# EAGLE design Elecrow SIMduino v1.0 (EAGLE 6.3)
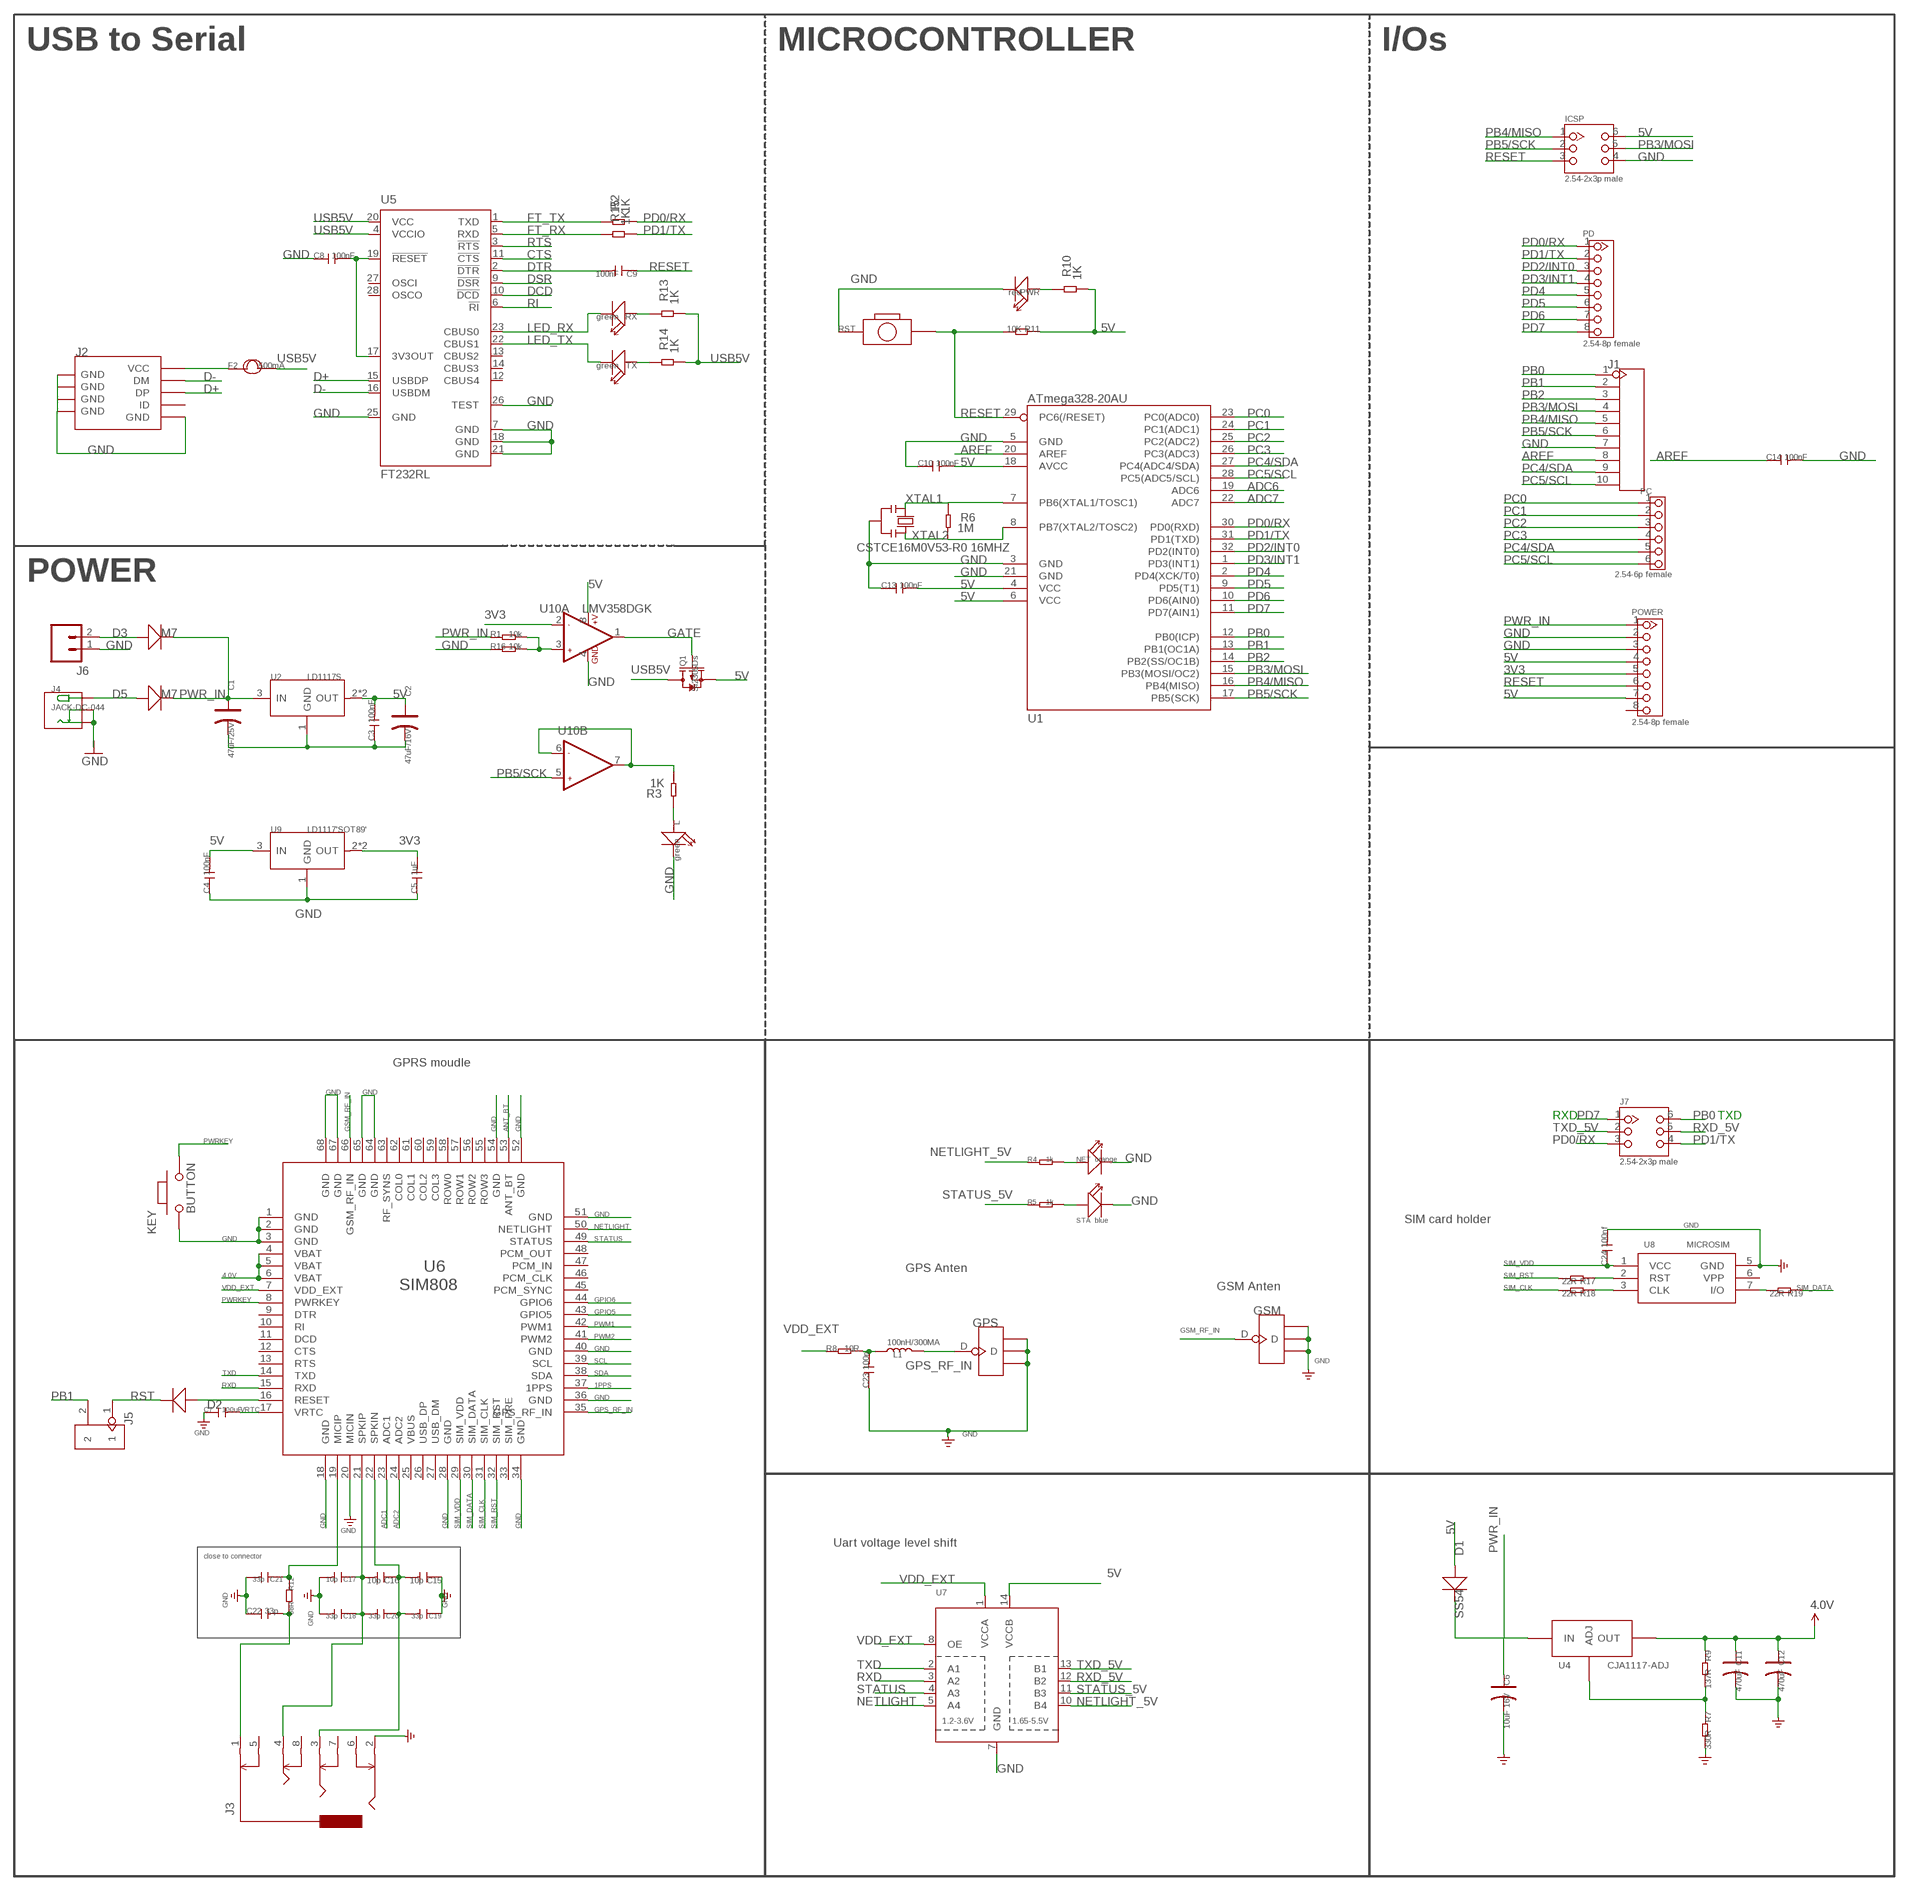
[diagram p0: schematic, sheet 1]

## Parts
C1  47uF/25V  CAP-AVX-C  [AVX-C]
C2  47uF/16V  CAP-AVX-A  [AVX-A]
C3  100nF  C-0603  [C0603]
C4  100nF  C-0603  [C0603]
C5  1uF  C-0603  [C0603]
C6  10uF 16V  CAP-AVX-A  [AVX-A]
C7  100uF  C-0805  [C0805]
C8  100nF  C-0603  [C0603]
C9  100nF  C-0603  [C0603]
C10  100nF  C-0603  [C0603]
C11  470uF  CAP-AVX-D  [AVX-D]
C12  470uF  CAP-AVX-D  [AVX-D]
C13  100nF  C-0603  [C0603]
C14  100nF  C-0603  [C0603]
C15  10p  C-0402  [C0402]
C16  10p  C-0402  [C0402]
C17  10p  C-0402  [C0402]
C18  33p  C-0402  [C0402]
C19  33p  C-0402  [C0402]
C20  33p  C-0402  [C0402]
C21  33p  C-0603  [C0603]
C22  33p  C-0603  [C0603]
C23  100n  C-0603  [C0603]
C24  100nf  C-0603  [C0603]
D1  SS54  D'MBRS240LT3'  [SMB]
D2  D'0805'  [SOD323]
D3  M7  D'SMA'  [D2010]
D5  M7  D'SMA'  [D2010]
F2  500mA  FUSE1206  [R1206]
GPS  ANTENNA-U-FL  [4P-U-FL]
GSM  ANTENNA-U-FL  [4P-U-FL]
ICSP  2.54-2x3p male  HEADER-2X3P-2.54  [2X3P-2.54]
J1  HEADER-10P-2.54  [10P-2.54]
J2  USB-MINIUSB-5P-STRONG  [MINI-SMD-5P]
J3  AUDIO-8P'PJ-3536-L6S'  [8P-3.5-SMD]
J4  JACK-DC-044  [DC-404]
J5  HEADER-2P-65/35MIL  [2P-2.54-65/35MIL]
J6  M02-JST-2MM-SMT  [JST-2-SMD]
J7  2.54-2x3p male  HEADER-2X3P-2.54  [2X3P-2.54]
KEY  BUTTON  PB157  [157SW]
L  green  LED'0603'  [LED-0603]
L1  100nH/300MA  L'0603'  [L0603]
NET  orange  LED'0603'  [LED-0603]
PC  2.54-6p female  HEADER-6P-65/35MIL  [6P-2.54-65/35MIL]
PD  2.54-8p female  HEADER-8P-2.54  [8P-2.54]
POWER  2.54-8p female  HEADER-8P-2.54  [8P-2.54]
PWR  red  LED'0603'  [LED-0603]
Q1  Si2305Ds  MOSFET-P'SI2323CDS/SI2305DS<BR>'  [SOT23]
R1  10k  R-0603  [R0603]
R2  1K  R-0603  [R0603]
R3  1K  R-0603  [R0603]
R4  1k  R-0603  [R0603]
R5  1k  R-0603  [R0603]
R6  1M  R-0603  [R0603]
R7  330R  R-0603  [R0603]
R8  10R  R-0603  [R0603]
R9  137R  R-0603  [R0603]
R10  1K  R-0603  [R0603]
R11  10K  R-0603  [R0603]
R12  68R  R-0603  [R0603]
R13  1K  R-0603  [R0603]
R14  1K  R-0603  [R0603]
R15  1K  R-0603  [R0603]
R16  10k  R-0603  [R0603]
R17  22R  R-0603  [R0603]
R18  22R  R-0603  [R0603]
R19  22R  R-0603  [R0603]
RST  BOTTON-2P-90D  [2P-7.62X3.56-90D]
RX  green  LED'0603'  [LED-0603]
STA  blue  LED'0603'  [LED-0603]
TX  green  LED'0603'  [LED-0603]
U1  ATmega328-20AU  ATMEGA168  [TQFP32]
U2  LD1117S  [SOT-223]
U4  CJA1117-ADJ  [SOT89]
U5  FT232RL  [SSOP28]
U6  SIM808  [SIM808]
U7  TXB0104PWR  [TSSOP14]
U8  MICROSIM  [MICROSIM]
U9  LD1117'SOT89'  [SOT89]
U10  LMV358DGK  [MSOP8]
Y2  CSTCE16M0V53-R0 16MHZ  RESONATORMU  [RESONATOR]

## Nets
1PPS: U6.37(1PPS)
3V3: C5.2 POWER.5 U9.2(OUT) U9.4(OUT) U10.2(A:-IN1)
4.0V: C11.+ C12.+ R9.1 U4.2(OUT) U4.4(OUT) U6.4(VBAT) U6.5(VBAT) U6.6(VBAT)
5V [usbvcc]: C2.+ C3.2 C4.2 C10.2 C13.2 D1.+ ICSP.6 POWER.4 POWER.7 Q1.2(S) R10.1 R11.1 U1.4(VCC) U1.6(VCC) U1.18(AVCC) U2.2(OUT) U2.TER(OUT) U7.14(VCCB) U9.3(IN) U10.8(A:+V)
ADC1: U6.23(ADC1)
ADC2: U6.24(ADC2)
ADC6: U1.19(ADC6)
ADC7: U1.22(ADC7)
ANT_BT: U6.53(ANT_BT)
AREF: C14.1 J1.8 U1.20(AREF)
CTS: U5.11(!CTS)
D+: J2.3(DP) U5.15(USBDP)
D-: J2.2(DM) U5.16(USBDM)
DCD: U5.10(!DCD)
DSR: U5.9(!DSR)
DTR: C9.2 U5.2(!DTR)
FT_RX: R15.2 U5.5(RXD)
FT_TX: R2.2 U5.1(TXD)
GATE: Q1.1(G) U10.1(A:OUT1)
GND: C1.- C2.- C3.1 C4.1 C5.1 C6.- C7.1 C8.1 C10.1 C11.- C12.- C13.1 C14.2 C15.1 C17.2 C18.2 C19.1 C21.2 C22.1 C23.1 C24.2 GPS.GND1 GPS.GND2 GPS.GND3 GSM.GND1 GSM.GND2 GSM.GND3 ICSP.4 J1.7 J2.5(GND) J2.GND@1(GND) J2.GND@2(GND) J2.GND@3(GND) J2.GND@4(GND) J3.2 J4.- J4.CDN J6.1 KEY.1 L.- NET.- POWER.2 POWER.3 PWR.- R7.2 R16.1 RST.P$1 STA.- U1.3(GND) U1.5(GND) U1.21(GND) U2.1(GND) U5.7(GND) U5.18(GND) U5.21(GND) U5.25(GND) U5.26(TEST) U6.1(GND) U6.2(GND) U6.3(GND) U6.18(GND) U6.20(MICIN) U6.28(GND) U6.34(GND) U6.36(GND) U6.40(GND) U6.51(GND) U6.52(GND) U6.54(GND) U6.64(GND) U6.65(GND) U6.67(GND) U6.68(GND) U7.7(GND) U8.5(GND) U9.1(GND) U10.4(A:GND) Y2.2
GPIO5: U6.43(GPIO5)
GPIO6: U6.44(GPIO6)
GPS_RF_IN: GPS.D L1.2 U6.35(GPS_RF_IN)
GSM_RF_IN: GSM.D U6.66(GSM_RF_IN)
LED_RX: RX.- U5.23(CBUS0)
LED_TX: TX.- U5.22(CBUS1)
N$1: D5.+ J4.+
N$2: R13.2 RX.+
N$3: L.+ R3.2
N$4: R5.2 STA.+
N$5: R3.1 U10.6(B:-IN2) U10.7(B:OUT2)
N$6: C8.2 U5.17(3V3OUT) U5.19(!RESET)
N$7: PWR.+ R10.2
N$8: R14.2 TX.+
N$9: F2.1 J2.1(VCC)
N$10: NET.+ R4.2
N$11: R18.1 U8.3(CLK)
N$12: R17.1 U8.2(RST)
N$13: C21.1 R12.1 U6.19(MICIP)
N$14: R1.2 R16.2 U10.3(A:+IN1)
N$15: C16.2 C17.1 C18.1 C20.2 J3.4 U6.21(SPKIP)
N$16: R19.2 U8.7(I/O)
N$17: R7.1 R9.2 U4.1(ADJ)
N$18: D2.+ U6.16(RESET)
N$19: C15.2 C16.1 C19.2 C20.1 J3.3 U6.22(SPKIN)
N$20: D3.+ J6.2
N$21: C23.2 L1.1 R8.2
N$30: C22.2 J3.1 R12.2
NETLIGHT: U6.50(NETLIGHT) U7.5(A4)
NETLIGHT_5V: R4.1 U7.10(B4)
PB0: J1.1 J7.6 U1.12(PB0(ICP))
PB1: J1.2 J5.2 U1.13(PB1(OC1A))
PB2: J1.3 U1.14(PB2(SS/OC1B))
PB3/MOSI: ICSP.5 J1.4 U1.15(PB3(MOSI/OC2))
PB4/MISO: ICSP.1 J1.5 U1.16(PB4(MISO))
PB5/SCK: ICSP.2 J1.6 U1.17(PB5(SCK)) U10.5(B:+IN2)
PC0: PC.1 U1.23(PC0(ADC0))
PC1: PC.2 U1.24(PC1(ADC1))
PC2: PC.3 U1.25(PC2(ADC2))
PC3: PC.4 U1.26(PC3(ADC3))
PC4/SDA: J1.9 PC.5 U1.27(PC4(ADC4/SDA))
PC5/SCL: J1.10 PC.6 U1.28(PC5(ADC5/SCL))
PD0/RX: J7.3 PD.1 R2.1 U1.30(PD0(RXD))
PD1/TX: J7.4 PD.2 R15.1 U1.31(PD1(TXD))
PD2/INT0: PD.3 U1.32(PD2(INT0))
PD3/INT1: PD.4 U1.1(PD3(INT1))
PD4: PD.5 U1.2(PD4(XCK/T0))
PD5: PD.6 U1.9(PD5(T1))
PD6: PD.7 U1.10(PD6(AIN0))
PD7: J7.1 PD.8 U1.11(PD7(AIN1))
PWM1: U6.42(PWM1)
PWM2: U6.41(PWM2)
PWR_IN: C1.+ C6.+ D1.- D3.- D5.- POWER.1 R1.1 U2.3(IN) U4.3(IN)
PWRKEY: KEY.2 U6.8(PWRKEY)
RESET: C9.1 ICSP.3 POWER.6 R11.2 RST.P$2 U1.29(PC6(/RESET))
RI: U5.6(!RI)
RST: D2.- J5.1
RTS: U5.3(!RTS)
RXD: U6.15(RXD) U7.3(A2)
RXD_5V: J7.5 U7.12(B2)
SCL: U6.39(SCL)
SDA: U6.38(SDA)
SIM_CLK: R18.2 U6.31(SIM_CLK)
SIM_DATA: R19.1 U6.30(SIM_DATA)
SIM_RST: R17.2 U6.32(SIM_RST)
SIM_VDD: C24.1 U6.29(SIM_VDD) U8.1(VCC)
STATUS: U6.49(STATUS) U7.4(A3)
STATUS_5V: R5.1 U7.11(B3)
TXD: U6.14(TXD) U7.2(A1)
TXD_5V: J7.2 U7.13(B1)
USB5V: F2.2 Q1.3(D) R13.1 R14.1 U5.4(VCCIO) U5.20(VCC)
VDD_EXT: R8.1 U6.7(VDD_EXT) U7.1(VCCA) U7.8(OE)
VRTC: C7.2 U6.17(VRTC)
XTAL1: R6.2 U1.7(PB6(XTAL1/TOSC1)) Y2.1
XTAL2: R6.1 U1.8(PB7(XTAL2/TOSC2)) Y2.3
Unconnected: J2.4(ID) J3.5 J3.6 J3.7 J3.8 POWER.8 U5.12(CBUS4) U5.13(CBUS2) U5.14(CBUS3) U5.27(OSCI) U5.28(OSCO) U6.9(DTR) U6.10(RI) U6.11(DCD) U6.12(CTS) U6.13(RTS) U6.25(VBUS) U6.26(USB_DP) U6.27(USB_DM) U6.33(SIM_PRE) U6.45(PCM_SYNC) U6.46(PCM_CLK) U6.47(PCM_IN) U6.48(PCM_OUT) U8.6(VPP)

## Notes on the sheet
- USB to Serial | MICROCONTROLLER | I/Os
- POWER
- GPRS moudle
- RXD | TXD
- SIM card holder
- GPS Anten
- GSM Anten
- Uart voltage level shift
- close to connector

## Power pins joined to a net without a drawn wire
COL0: U6.62(COL0)
COL1: U6.61(COL1)
COL2: U6.60(COL2)
COL3: U6.59(COL3)
RF_SYNS: U6.63(RF_SYNS)
ROW0: U6.58(ROW0)
ROW1: U6.57(ROW1)
ROW2: U6.56(ROW2)
ROW3: U6.55(ROW3)

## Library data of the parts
C1 C2 = Discrete:CAP*: Electrolytic Capacitors,Tantalum Capacitors and Super Capacitors
C3-C5 C7-C10 C13-C24 = Discrete:C*: Ceramic Capacitors
C6 C11 C12 = Common:CAP*
D1-D3 D5 = Discrete:D*
F2 = Discrete:FUSE
GPS GSM = Connector:ANTENNA-U-FL
ICSP J7 = Connector:HEADER-2X3P
J1 = Connector:HEADER-10P
J2 = Connector:USB-MINIUSB-5P
J3 = template:AUDIO-8P
J4 = Connector:JACK-DC-044
J5 = Connector:HEADER-2P
J6 = SparkFun:M02: Header 2
KEY = MySMD:PB157
L NET PWR RX STA TX = Discrete:LED*
L1 = Discrete:L*
PC = Connector:HEADER-6P
PD POWER = Connector:HEADER-8P
Q1 = Discrete:MOSFET-P
R1-R19 = Discrete:R*
RST = Discrete:BOTTON-2P
U1 = IC:ATMEGA168
U2 U9 = IC:LD1117: Low Drop Fixed And Adjustable Positive Voltage Regulators http://www.datasheetcatalog.org/datasheet/SGSThomsonMicroelectronics/mXuqtqv.pdf
U4 = IC:CJA1117-ADJ
U5 = IC_SMD:FT232R: Source: http://www.ftdichip.com/Documents/DataSheets/DS_FT232R_v104.pdf
U6 = moudle:SIM808
U7 = adafruit:TXB0104PWR: 4-Bit Bi-Directional Level Shifter 1.2V-3.6V (VCCA) to 1.65V-5.5V (VCCB) bi-directional level shifter with auto direction sensing. Max data rate - VCCA 1.8V: 20Mbps (50ns), VCCA 3.3V: 100Mbps (10ns) Digikey: 296-21929-1-ND
U8 = Connector:MICROSIM
U10 = IC:LMV358: General purpose LOW Voltage, Rail-to-Rail Output Amplifiers http://www.fairchildsemi.com/ds/LM/LMV358.pdf
Y2 = SmartPrj:RESONATOR

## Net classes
0 default: width 0.203 mm
1 power: width 0.61 mm, drill 0.61 mm, clearance 0.254 mm
2 gnd: width 0.305 mm, drill 0.559 mm, clearance 0.254 mm
3 usbvcc: width 0.508 mm, drill 0.61 mm, clearance 0.254 mm

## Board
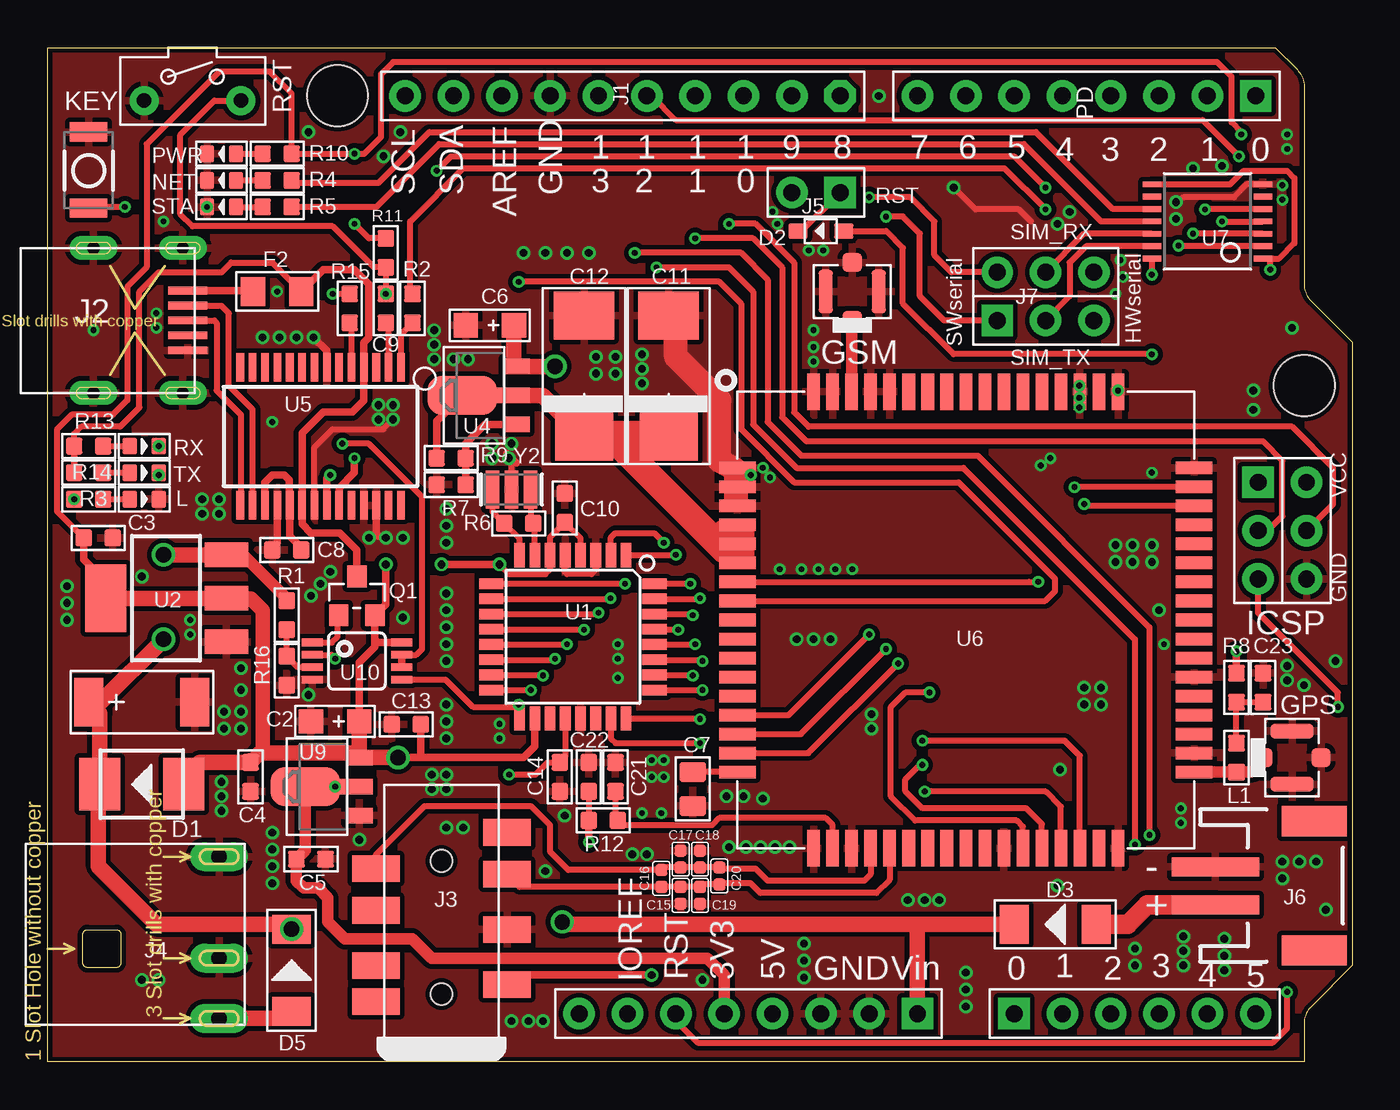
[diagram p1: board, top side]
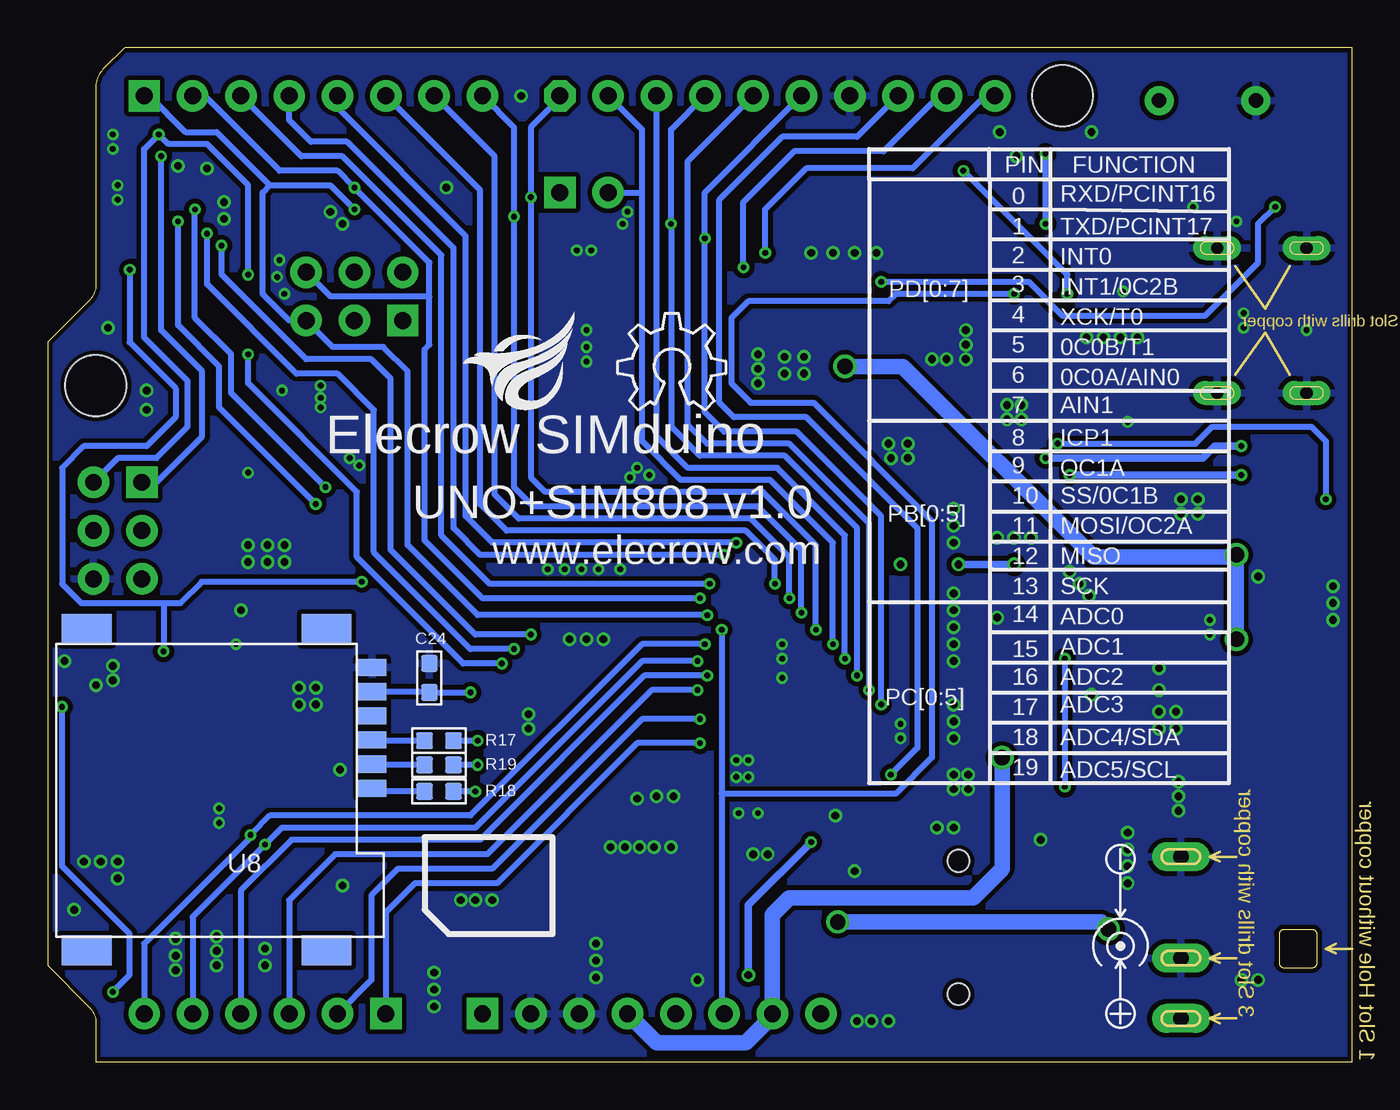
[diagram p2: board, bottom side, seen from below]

Size 68.58 x 53.34 mm. Coordinates in mm from the lower left corner, seen from the top.
Outline: 0,0 0,53.34 64.52,53.34 65.67,52.19 arc-45 66.04,51.29 66.04,40.91 arc45 66.41,40.01 68.58,37.85 68.58,5.08 66.41,2.91 arc45 66.04,2.01 66.04,0 0,0
Copper layers (1*16): Top 0.035mm / dielectric 1.5mm / Bottom 0.035mm
Design rules "Elecrow_2-layer_eagle_rule": minimum track width 6mil, minimum drill 12mil, track to track 6mil, track to pad 6mil, pad to pad 6mil, via to via 6mil, smd to smd 0mil, copper to edge 10mil, drill to drill 10mil, minimum pad ring 10mil, minimum via ring 6mil, stop-mask expansion 2mil, vias tented up to drill 100mil, thermal gap 10mil
Holes 3.2 mm at 15.24,50.8 66.04,35.56
tRestrict: area 21.7,32.4 to 21.8,34; area 44.2,24.4 to 44.6,24.6

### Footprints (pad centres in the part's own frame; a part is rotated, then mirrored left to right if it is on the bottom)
AVX-C = smd 1.524 x 2.54: + -2.794,0; - 2.794,0
AVX-A = smd 1.27 x 1.27: + -1.27,0; - 1.27,0
C0603 = smd 0.889 x 0.889: 1 -0.762,0; 2 0.762,0
C0805 = smd 1.016 x 1.397: 1 -0.889,0; 2 0.889,0
AVX-D = smd 2.54 x 3.048: + -3.175,0 | smd 2.54 x 3.175: - 3.175,0
C0402 = smd 0.635 x 0.635: 1 -0.445,0; 2 0.445,0
SMB = smd 2.159 x 2.743: + -2.21,0; - 2.21,0
SOD323 = smd 1 x 0.8: + -1.2,0; - 1.2,0
D2010 = smd 1.524 x 2.032: + -2.159,0; - 2.159,0
R1206 = smd 1.27 x 1.524: 1 -1.27,0; 2 1.27,0
4P-U-FL = smd 1.016 x 1.016: D -1.524,0; GND3 1.524,0 | smd 2.286 x 0.762: GND1 0,1.397; GND2 0,-1.397
2X3P-2.54 = drill 0.889 pad 1.651 square: 1 -1.27,2.54 | drill 0.889 pad 1.651: 2 -1.27,0; 3 -1.27,-2.54; 4 1.27,-2.54; 5 1.27,0; 6 1.27,2.54
10P-2.54 = drill 0.889 pad 1.651 octagon: 1 0,11.43 | drill 0.889 pad 1.651: 2 0,8.89; 3 0,6.35; 4 0,3.81; 5 0,1.27; 6 0,-1.27; 7 0,-3.81; 8 0,-6.35; 9 0,-8.89; 10 0,-11.43
MINI-SMD-5P = smd 2.032 x 0.406: 1 0.381,-1.575; 2 0.381,-0.787; 3 0.381,0; 4 0.381,0.787; 5 0.381,1.575 | drill 0.635 pad 1.27 long: GND@1 0.635,3.81; GND@2 5.334,3.81; GND@3 5.334,-3.81; GND@4 0.635,-3.81
8P-3.5-SMD = smd 1.4 x 2.5: 1 2.8,-3.45; 2 5.7,-3.45; 3 8.6,-3.45; 4 8.9,3.45; 5 1.9,3.45; 6 3.8,3.45; 7 6.7,3.45; 8 10.8,-3.45 | hole 1.149: 2.3,0; 9.3,0
DC-404 = drill 0.813 pad 1.524 long: + 3.175,10.16; - -5.334,10.16; CDN 0,10.16
2P-2.54-65/35MIL = drill 0.889 pad 1.651 square: 1 0,1.27 | drill 0.889 pad 1.651: 2 0,-1.27
JST-2-SMD = smd 1 x 4.6: 1 -1,-3.7; 2 1,-3.7 | smd 1.6 x 3.4: NC1 -3.4,1.5; NC2 3.4,1.5
157SW = smd 1.016 x 1.981: 1 0,0; 2 4,0
LED-0603 = smd 0.762 x 0.889: + -0.762,0; - 0.762,0
L0603 = smd 0.889 x 0.889: 1 -0.762,0; 2 0.762,0
6P-2.54-65/35MIL = drill 0.889 pad 1.651 square: 1 0,6.35 | drill 0.889 pad 1.651: 2 0,3.81; 3 0,1.27; 4 0,-1.27; 5 0,-3.81; 6 0,-6.35
8P-2.54 = drill 0.889 pad 1.651 square: 1 0,8.89 | drill 0.889 pad 1.651: 2 0,6.35; 3 0,3.81; 4 0,1.27; 5 0,-1.27; 6 0,-3.81; 7 0,-6.35; 8 0,-8.89
SOT23 = smd 1.016 x 1.143: 1 -0.95,-1.016; 2 0.95,-1.016; 3 0,1.016
R0603 = smd 0.889 x 0.889: 1 -0.762,0; 2 0.762,0
2P-7.62X3.56-90D = drill 0.762 pad 1.524: P$1 0,2.54; P$2 0,-2.54
TQFP32 = smd 1.27 x 0.559: 1 -4.293,2.8; 2 -4.293,2; 3 -4.293,1.2; 4 -4.293,0.4; 5 -4.293,-0.4; 6 -4.293,-1.2; 7 -4.293,-2; 8 -4.293,-2.8; 17 4.293,-2.8; 18 4.293,-2; 19 4.293,-1.2; 20 4.293,-0.4; 21 4.293,0.4; 22 4.293,1.2; 23 4.293,2; 24 4.293,2.8 | smd 0.559 x 1.27: 9 -2.8,-4.293; 10 -2,-4.293; 11 -1.2,-4.293; 12 -0.4,-4.293; 13 0.4,-4.293; 14 1.2,-4.293; 15 2,-4.293; 16 2.8,-4.293; 25 2.8,4.293; 26 2,4.293; 27 1.2,4.293; 28 0.4,4.293; 29 -0.4,4.293; 30 -1.2,4.293; 31 -2,4.293; 32 -2.8,4.293
SOT-223 = smd 1.27 x 2.286: 1 -2.286,-3.175; 2 0,-3.175; 3 2.286,-3.175 | smd 3.556 x 2.159: TER 0,3.175
SOT89 = smd 0.8 x 1.4: 1 -1.524,-1.905; 3 1.524,-1.905 | smd 0.8 x 1.9: 2 0,-1.651 | smd 2.032 x 3.65: 4 0,0.94
SSOP28 = smd 0.4 x 1.5: 1 -4.225,-3.625; 2 -3.575,-3.625; 3 -2.925,-3.625; 4 -2.275,-3.625; 5 -1.625,-3.625; 6 -0.975,-3.625; 7 -0.325,-3.625; 8 0.325,-3.625; 9 0.975,-3.625; 10 1.625,-3.625; 11 2.275,-3.625; 12 2.925,-3.625; 13 3.575,-3.625; 14 4.225,-3.625; 15 4.225,3.625; 16 3.575,3.625; 17 2.925,3.625; 18 2.275,3.625; 19 1.625,3.625; 20 0.975,3.625; 21 0.325,3.625; 22 -0.325,3.625; 23 -0.975,3.625; 24 -1.625,3.625; 25 -2.275,3.625; 26 -2.925,3.625; 27 -3.575,3.625; 28 -4.225,3.625
SIM808 = smd 1.93 x 0.66: 1 -10.349,7.238; 2 -10.349,6.238; 3 -10.349,5.238; 4 -10.349,4.238; 5 -10.349,3.238; 6 -10.349,2.238; 7 -10.349,1.238; 8 -10.349,0.238; 9 -10.349,-0.762; 10 -10.349,-1.762; 11 -10.349,-2.762; 12 -10.349,-3.762; 13 -10.349,-4.762; 14 -10.349,-5.762; 15 -10.349,-6.762; 16 -10.349,-7.762; 17 -10.349,-8.762; 35 13.651,-8.762; 36 13.651,-7.762; 37 13.651,-6.762; 38 13.651,-5.762; 39 13.651,-4.762; 40 13.651,-3.762; 41 13.651,-2.762; 42 13.651,-1.762; 43 13.651,-0.762; 44 13.651,0.238; 45 13.651,1.238; 46 13.651,2.238; 47 13.651,3.238; 48 13.651,4.238; 49 13.651,5.238; 50 13.651,6.238; 51 13.651,7.238 | smd 0.66 x 1.93: 18 -6.349,-12.762; 19 -5.349,-12.762; 20 -4.349,-12.762; 21 -3.349,-12.762; 22 -2.349,-12.762; 23 -1.349,-12.762; 24 -0.349,-12.762; 25 0.651,-12.762; 26 1.651,-12.762; 27 2.651,-12.762; 28 3.651,-12.762; 29 4.651,-12.762; 30 5.651,-12.762; 31 6.651,-12.762; 32 7.651,-12.762; 33 8.651,-12.762; 34 9.651,-12.762; 52 9.651,11.238; 53 8.651,11.238; 54 7.651,11.238; 55 6.651,11.238; 56 5.651,11.238; 57 4.651,11.238; 58 3.651,11.238; 59 2.651,11.238; 60 1.651,11.238; 61 0.651,11.238; 62 -0.349,11.238; 63 -1.349,11.238; 64 -2.349,11.238; 65 -3.349,11.238; 66 -4.349,11.238; 67 -5.349,11.238; 68 -6.349,11.238
TSSOP14 = smd 0.305 x 0.991: 1 -1.95,-2.918; 2 -1.3,-2.918; 3 -0.65,-2.918; 4 0,-2.918; 5 0.65,-2.918; 6 1.3,-2.918; 7 1.95,-2.918; 8 1.95,2.918; 9 1.3,2.918; 10 0.65,2.918; 11 0,2.918; 12 -0.65,2.918; 13 -1.3,2.918; 14 -1.95,2.918
MICROSIM = smd 1.5 x 0.9: 1 -0.8,2.5; 2 -0.8,5.04; 3 -0.8,7.58; 5 -0.8,1.23; 6 -0.8,3.77; 7 -0.8,6.31 | smd 2.61 x 1.56: P$1 1.6,-0.8; P$2 14.2,-0.8; P$3 14.2,16.1; P$4 1.6,16.1
MSOP8 = smd 0.4 x 1.1: 1 -0.975,-2.35; 2 -0.325,-2.35; 3 0.325,-2.35; 4 0.975,-2.35; 5 0.975,2.35; 6 0.325,2.35; 7 -0.325,2.35; 8 -0.975,2.35
RESONATOR = smd 0.7 x 2: 1 -1,0; 2 0,0; 3 1,0

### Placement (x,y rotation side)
C1  4.95,18.92 0 top
C2  15.11,17.91 180 top
C3  2.67,27.56 180 top
C4  10.67,14.99 90 top
C5  13.84,10.67 180 top
C6  23.24,38.73 180 top
C7  33.91,14.35 90 top
C8  12.57,26.92 0 top
C9  17.78,39.62 270 top
C10  27.18,29.13 270 top
C11  32.64,36.07 90 top
C12  28.19,36.07 90 top
C13  18.85,17.75 0 top
C14  26.92,14.99 270 top
C15  33.27,8.76 90 top
C16  32.26,9.65 90 top
C17  33.27,10.67 90 top
C18  34.29,10.67 90 top
C19  34.29,8.76 90 top
C20  35.31,9.78 90 top
C21  29.84,14.99 90 top
C22  28.45,14.99 270 top
C23  63.88,19.68 270 top
C24  48.51,20.19 90 bottom
D1  4.95,14.61 180 top
D2  40.64,43.69 180 top
D3  52.96,7.24 180 top
D5  12.83,4.83 90 top
F2  12.06,40.51 0 top
GPS  65.41,16 0 top
GSM  42.29,40.51 90 top
ICSP  64.9,27.94 0 top
J1  30.23,50.8 270 top
J2  7.75,38.99 180 top
J3  20.7,1.27 90 top
J4  -1.14,5.46 270 top
J5  40.39,45.72 270 top
J6  65.07,9.27 270 top
J7  52.45,40.26 90 top
KEY  2.16,48.9 270 top
L  5.08,29.59 0 top
L1  62.48,16 270 top
NET  9.14,46.35 180 top
PC  57.15,2.54 90 top
PD  54.61,50.8 270 top
POWER  36.83,2.54 270 top
PWR  9.14,47.75 180 top
Q1  16.26,24.51 0 top
R1  12.57,23.5 270 top
R2  19.18,39.62 270 top
R3  2.16,29.59 0 top
R4  12.06,46.35 180 top
R5  12.06,44.96 180 top
R6  24.77,28.32 0 top
R7  21.21,30.35 180 top
R8  62.48,19.68 270 top
R9  21.21,31.75 0 top
R10  12.06,47.75 180 top
R11  17.78,42.55 270 top
R12  29.21,12.7 180 top
R13  2.16,32.38 0 top
R14  2.16,30.99 0 top
R15  15.88,39.62 270 top
R16  12.57,20.57 90 top
R17  48.01,16.89 0 bottom
R18  48.01,14.22 0 bottom
R19  48.01,15.62 180 bottom
RST  7.62,50.55 90 top
RX  5.08,32.38 0 top
STA  9.14,44.96 180 top
TX  5.08,30.99 0 top
U1  27.61,22.35 270 top
U2  6.22,24.38 90 top
U4  22.73,35.05 90 top
U5  14.35,32.89 180 top
U6  46.61,24 0 top
U7  60.96,44.2 90 top
U8  52.32,21.97 180 bottom
U9  14.48,14.48 90 top
U10  16.26,21.08 270 top
U$1  [OSHW_6X200_NOTEXT]  38.61,34.29 0 bottom
U$2  [ELECROW_NEW_4]  46.74,34.29 0 bottom
Y2  24.38,30.1 180 top

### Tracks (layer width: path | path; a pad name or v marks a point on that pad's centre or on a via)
3V3  (via drill 0.3)
  Top 0.305: U10.2 14.91,21.41 v15.11,21.21
  Top 0.61: U9.2 v15.11,14.48 U9.4 13.54,11.12 C5.2 13.08,9.53 13.46,9.14 14.22,9.14 14.73,8.64 14.73,7.37 15.62,6.48 19.18,6.48 20.19,5.46 34.67,5.46 35.56,4.57 POWER.5
  Bottom 0.305: v15.11,21.21 v15.11,14.48
4.0V
  Top 0.305: U4.4 U4.2
  Top 0.406: U6.6 U6.5 36.26,26.61 36.7,26.16 36.96,26.16 36.96,26.67 | R9.1 20.45,33.71 U4.4 | U6.4 36.4,28.24 36.7,27.94 | 36.7,27.94 36.96,27.69 | 36.96,27.69 36.96,27.94 36.7,27.94 | 36.96,27.69 36.96,26.67 | 36.96,26.67 36.45,26.67 36.45,27.94 36.32,27.94 36.32,27.69 | 36.32,27.69 36.7,27.69 36.7,26.92 | 36.32,27.69 35.56,27.69
  Top 0.813: 27.18,32.77 28.07,32.77 C12.+ 26.04,35.05 U4.2
  Top 1.422: C12.+ 29.59,32.89 35.56,26.92 35.56,27.69 35.56,27.81
  Top 1.676: C12.+ C11.+
5V  (via drill 0.3, 0.41, 0.81)
  Top 0.305: v23.75,26.16 24.26,25.65 26.16,25.65 26.42,25.91 U1.6 26.41,27.6 C10.2 28.01,27.54 U1.4 | v62.74,48.77 62.74,48.9 62.23,49.4 62.23,51.82 61.47,52.58 18.16,52.58 17.53,51.94 17.53,48.64 16.64,47.75 v16.13,47.75 R10.1 12.83,50.93 11.68,52.07 9.02,52.07 5.21,48.26 5.21,41.78 4.19,40.77 4.19,34.8 3.43,34.04 1.27,34.04 0.51,33.27 0.51,28.96 C3.2 | R11.1 16.89,43.31 v16.13,44.07 | U7.14 v58.04,41.41 v58.04,41.4
  Top 0.406: C2.+ 16.38,21 17.21,21.82 17.21,22.23 | U2.TER 3.05,25.27 1.91,26.42 C3.2 | v23.75,26.16 v20.7,26.16 | 19.56,16 25.02,16 25.61,16.59 U1.18 | 19.56,16 v18.41,16 | C13.2 19.61,16.05 19.56,16 | v17.78,26.16 17.78,24.07 Q1.2 17.21,22.23 | U10.8 17.37,22.06 17.21,22.23
  Top 0.762: U2.2 10.67,24.38 11.3,23.75 11.3,16.38 11.05,16.13 C4.2
  Top 0.813: 10.59,15.82 C4.2 8,15.75 7.16,14.91 D1.+ | U9.3 C2.+ | U2.TER U2.2 | 11.05,16.13 11.18,16.26 16.13,16.26 U9.3 | U9.3 v18.41,16
  Bottom 0.305: v16.13,44.07 v16.13,47.75 | v58.04,41.4 58.04,46.1 60.2,48.26 62.23,48.26 v62.74,48.77 63.5,48.01 63.5,38.1 61.21,35.81 61.21,33.4 62.87,31.75 64.9,31.75 ICSP.6
  Bottom 0.406: v20.7,26.16 v17.78,26.16
  Bottom 0.61: POWER.7 30.48,2.41
  Bottom 0.813: v18.41,16 18.41,10.16 19.94,8.64 29.59,8.64 30.48,7.75 POWER.7 | 30.48,2.41 31.88,1.02 36.58,1.02 POWER.4
AREF  (via drill 0.3)
  Top 0.305: U1.20 27.21,16.09 C14.1 26.29,15.75 25.65,15.11 v24.26,15.11
  Bottom 0.305: J1.8 26.04,48.64 29.97,48.64 33.27,45.34 33.27,34.67 32.51,33.91 28.7,33.91 22.86,28.07 22.86,16.51 v24.26,15.11
D+
  Top 0.305: J2.3 8.76,38.99 8.89,38.86 8.89,35.31 10.16,34.04 10.16,29.3 U5.15
D-
  Top 0.305: U5.16 10.78,34.31 9.53,35.56 9.53,39.37 9.14,39.75 7.39,39.75 J2.2
DTR
  Top 0.305: U5.2 17.93,38.72 C9.2
FT_RX
  Top 0.305: U5.5 15.98,38.76 R15.2
FT_TX
  Top 0.305: U5.1 18.58,38.26 R2.2
GATE
  Top 0.305: U10.1 14.95,22.06 15.24,22.35 15.24,23.43 Q1.1
GND  (via drill 0.3, 0.41)
  Top 0.305: U7.7 63.04,46.15 62.36,45.47 59.69,45.47 v59.31,45.21 | U6.52 v56.26,35.3 v56.26,35.31 | v54.23,34.92 54.23,34.76 U6.54 | U1.3 28.81,25.89 28.57,25.65 27.3,25.65 27.18,25.78 27.18,26.61 U1.5 | Y2.2 24.38,31.75 24.26,31.88 v24.26,31.75 | U5.21 14.03,32.31 14.99,33.27 17.65,33.27 v18.16,33.78 | 51.69,44.2 51.05,44.83 48.77,44.83 v47.62,45.97
  Top 0.406: U5.18 12.08,27.32 C8.1 | U5.26 17.28,27.68 v17.78,27.56 | U5.7 14.68,37.39 v13.97,38.1 | 24.64,31.5 24.26,31.88 24.13,32
  Top 1.27: 36.2,29.59 36.2,31.11 35.31,31.62 35.31,34.8 33.02,37.08 33.02,39.37
  other vias: 14.86,25.78 20.95,24.64 20.95,17.91 20.95,15.11 13.72,19.3 11.81,33.66 9.02,29.59 20.32,37.72 5.71,39.37 5.71,38.61 12.06,40.51 8.38,44.96 6.1,44.2 4.95,25.53 2.41,38.48 40.26,37.59 38.35,44.07 20.95,28.19 18.67,23.37 29.97,21.21 29.97,20.19 23.75,17.02 23.75,17.78 65.15,20.83 58.42,23.75 58.67,21.97 58.04,30.99 65.15,48.01 65.41,38.61 65.15,48.77 61.72,47.12 40.26,38.48 40.26,36.83 40.77,42.67 40.01,42.67 54.23,35.56 54.23,34.42 52.2,31.37 63.37,35.31 63.37,34.29 35.69,13.97 35.81,11.3 37.47,11.3 48.26,4.7 46.86,8.51 38.48,25.91 39.62,25.91 20.95,17.02 20.95,18.8 1.02,25.02 1.02,24.13 20.95,27.3 7.49,23.24 7.49,22.48 10.16,19.56 10.16,18.41 31.24,37.21 31.24,36.45 31.24,35.69 29.84,37.08 29.84,36.2 20.32,36.96 23.37,31.75 24.38,32.51 23.37,32.51 28.83,37.08 28.83,36.2 20.95,29.08 20.95,23.75 20.95,22.86 18.67,27.56 16.89,27.56 13.08,38.1 12.19,38.1 11.3,38.1 28.45,42.55 27.3,42.55 26.16,42.55 25.02,42.55 20.32,38.48 21.34,36.96 22.1,36.96 17.4,33.78 18.16,34.54 17.4,34.54 20.95,21.97 20.95,21.08 14.35,25.15 13.84,24.51 10.16,20.7 10.16,17.53 9.27,18.41 9.27,17.53 9.14,14.73 9.14,13.97 9.14,13.21 11.81,12.06 11.81,11.18 11.81,10.29 1.02,23.24 9.02,28.83 8.13,29.59 8.13,28.83 31.75,15.88 32.38,15.88 31.75,14.99 32.38,14.99 38.23,11.3 38.99,11.3 43.31,18.29 43.31,17.53 55.37,19.68 54.48,19.68 55.37,18.8 54.48,18.8 59.69,6.6 57.15,5.97 48.26,3.81 48.26,2.92 46.1,8.51 45.21,8.51 58.04,27.18 57.02,27.18 56.13,27.18 58.04,26.29 57.02,26.29 56.13,26.29 40.51,25.91 41.4,25.91 42.29,25.91 29.97,21.97 20.19,15.11 60.2,46.99 59.31,44.32 53.21,15.37 36.58,13.97 37.59,13.84 5.84,4.32 41.15,22.23 65.79,10.54 66.67,10.54 64.9,10.54 64.9,9.65 65.15,20.07 36.7,11.3 26.16,10.03 31.5,10.92 30.73,10.92 27.18,12.95 20.95,14.35 20.19,14.35 4.95,4.32 34.42,4.32 53.72,44.7 32.26,13.08 31.24,13.08 17.65,47.62 18.54,48.9 13.72,48.9 39.75,5.33 66.04,19.81 67.69,21.08 67.18,8 40.26,22.23 39.37,22.23 43.69,50.8 56.39,42.16 56.13,40.39 56.52,41.27 53.09,44.07 59.69,5.84 57.15,5.08 61.85,6.48 61.85,5.59 61.85,4.83 59.69,5.08 37.59,31.24 37.97,30.73 36.96,30.86 38.1,44.7 59.56,13.34 59.56,12.57 64.9,46.1 64.9,45.34 52.7,31.75 39.75,6.22 39.75,4.45 25.27,2.16 24.38,2.16 26.04,2.16 21.84,12.32 20.95,12.32 16.38,11.68 11.81,9.4 53.09,9.27
  pour Top (isolate 0.254, rank 6): 0,53.34 68.58,53.34 68.58,0 0,0
  pour Bottom (isolate 0.254, rank 6): 0,53.34 68.58,53.34 68.58,0 0,0
GPS_RF_IN
  Top 0.61: U6.35 L1.2 63.12,15.24 arc90 GPS.D
GSM_RF_IN
  Top 0.61: U6.66 42.26,38.96 GSM.D
LED_RX  (via drill 0.3)
  Top 0.406: U5.23 15.33,30.18 16.13,30.99 v16.13,31.75
  Bottom 0.406: v16.13,31.75 7.87,31.75 7.24,32.38 RX.-
  other vias: 5.84,32.38
LED_TX  (via drill 0.3)
  Top 0.406: v5.84,30.86 5.97,30.86 TX.- | U5.22 14.68,30.68 v14.86,30.86
  Bottom 0.406: v14.86,30.86 v5.84,30.86
N$1
  Top 0.813: J4.+ 12.45,2.29 D5.+
N$2
  Top 0.305: R13.2 RX.+
N$3
  Top 0.305: R3.2 L.+
N$4
  Top 0.305: STA.+ R5.2
N$5  (via drill 0.3)
  Top 0.305: U10.7 19.38,21.41 19.68,21.72 19.68,29.72 16.89,32.51 v15.49,32.51
  Top 0.406: U10.7 U10.6
  Bottom 0.305: v15.49,32.51 8.26,32.51 7.37,33.4 2.16,33.4 1.4,32.64 R3.1
  other vias: 1.4,29.59
N$6
  Top 0.406: U5.17 11.43,30.48 11.81,30.86 12.45,30.86 12.7,30.61 12.7,29.29 U5.19 12.73,27.66 13.34,27.05 C8.2
N$7
  Top 0.305: PWR.+ R10.2
N$8
  Top 0.305: R14.2 TX.+
N$9
  Top 0.406: J2.1 10.74,40.56 F2.1
N$10
  Top 0.305: NET.+ R4.2
N$11
  Bottom 0.305: R18.1 51.36,14.22 U8.3
N$12
  Bottom 0.305: R17.1 51.48,16.89 U8.2
N$13
  Top 0.305: C21.1 29.84,12.83 R12.1 30.23,12.45 34.92,12.45 35.31,12.83 40.89,12.83 41.26,12.46 U6.19
N$14
  Top 0.305: U10.3 13.15,20.76 R16.2 R1.2
N$15
  Top 0.305: J3.4 17.25,10.9 19.81,13.46 25.4,13.46 26.42,12.45 26.42,11.05 27.37,10.1 C16.2 32.38,10.22 C17.1 C18.1 C20.2 35.37,10.16 37.21,10.16 37.85,9.53 42.93,9.53 43.26,9.86 U6.21
N$16
  Bottom 0.305: R19.2 51.48,15.62 U8.7
N$17
  Top 0.406: R7.1 R9.2 21.97,32.51 22.99,33.53 U4.1
N$18  (via drill 0.3)
  Top 0.305: D2.+ 44.07,43.69 44.96,42.8 44.96,39.88 47.62,37.21 v58.04,37.21 | U6.16 39.99,16.24 v44.7,20.95
  Bottom 0.305: v44.7,20.95 46.74,20.95 52.32,26.54 52.32,29.97 58.04,35.69 v58.04,37.21
N$19
  Top 0.305: J3.3 24.81,9.21 C16.1 C15.2 C19.2 34.42,9.34 C20.1 35.37,9.4 36.96,9.4 37.47,8.89 43.56,8.89 44.26,9.59 U6.22
N$20
  Top 1.016: J6.2 57.8,8.27 56.77,7.24 D3.+
N$21
  Top 0.305: L1.1 R8.2 C23.2
N$30  (via drill 0.3, 0.41)
  Top 0.305: C22.2 R12.2
  Top 0.406: v28.45,11.56 R12.2 | v31.75,4.57 24.65,4.57 J3.1
  Bottom 0.406: v31.75,4.57 31.75,8.26 v28.45,11.56
NETLIGHT  (via drill 0.3)
  Top 0.305: 60.96,44.83 v60.83,44.83 60.85,44.85 U7.5 | U6.50 v53.99,30.24 v53.98,30.23
  Bottom 0.305: v60.83,44.83 60.83,39.12 58.93,37.21 58.93,35.18 v53.98,30.23
NETLIGHT_5V
  Top 0.305: R4.1 12.95,46.23 17.4,46.23 20.07,48.9 51.94,48.9 55.99,44.85 U7.10
PB0  (via drill 0.3)
  Top 0.305: U1.12 28.18,22.75 v28.19,22.73 | J7.6 47.5,41.53 46.61,42.42 46.61,44.2 45.34,45.47 v43.18,45.47
  Bottom 0.305: v28.19,22.73 28.19,27.18 30.99,29.97 42.42,29.97 43.18,30.73 v43.18,45.47 43.18,49.15 41.66,50.67 J1.1
PB1  (via drill 0.3)
  Top 0.305: U1.13 27.29,21.95 v27.3,21.97
  Bottom 0.305: v27.3,21.97 27.3,27.3 30.61,30.61 35.31,30.61 37.34,32.64 37.34,45.72 | 37.34,45.72 37.34,49.02 J1.2 | J5.2 37.34,45.72
PB2  (via drill 0.3)
  Top 0.305: U1.14 26.61,21.15 v26.67,21.21
  Bottom 0.305: v26.67,21.21 26.67,27.69 30.23,31.24 34.92,31.24 36.58,32.89 J1.3
PB3/MOSI  (via drill 0.3)
  Top 0.305: U1.15 26,20.35 v26.04,20.32 | ICSP.5 67.56,29.34 67.56,31.24 65.41,33.4 40.01,33.4 39.24,34.16 39.24,42.04 37.21,44.07 v35.81,44.07
  Bottom 0.305: v26.04,20.32 26.04,28.07 29.84,31.88 34.29,31.88 35.81,33.4 v35.81,44.07 35.81,49.02 J1.4
PB4/MISO  (via drill 0.3)
  Top 0.305: U1.16 v25.39,19.55 v25.4,19.56 | v62.61,47.62 60.71,49.53 33.02,49.53 31.75,50.8 J1.5
  Bottom 0.305: v25.4,19.56 25.4,28.32 29.59,32.51 33.91,32.51 34.92,33.53 34.92,47.37 J1.5 | v62.61,47.62 62.61,38.48 60.45,36.32 60.45,32.89 62.87,30.48 ICSP.1
PB5/SCK  (via drill 0.3)
  Top 0.305: U1.17 24.77,18.1 v24.77,18.8 24.64,18.67 22.35,18.67 20.91,20.11 U10.5 | ICSP.2 64.14,27.94 64.9,28.7 64.9,31.62 63.88,32.64 39.88,32.64 38.61,33.91 38.61,41.78 37.08,43.31 v34.04,43.31
  Bottom 0.305: v24.77,18.8 24.77,28.7 29.21,33.15 33.02,33.15 34.04,34.16 v34.04,43.31 34.04,45.72 J1.6
PC0  (via drill 0.3)
  Top 0.305: U1.23 29.61,17 29.84,16.76 v34.29,16.76
  Bottom 0.305: v34.29,16.76 37.59,16.76 44.96,9.4 49.28,9.4 50.8,7.87 PC.1
PC1  (via drill 0.3)
  Top 0.305: U1.24 34.27,18.06 v34.29,18.03
  Bottom 0.305: v34.29,18.03 37.34,18.03 45.21,10.16 50.16,10.16 51.56,8.76 51.56,4.32 PC.2
PC2  (via drill 0.3)
  Top 0.305: U1.25 v34.41,19.55 v34.42,19.56
  Bottom 0.305: v34.42,19.56 36.83,19.56 45.47,10.92 53.47,10.92 55.88,8.51 PC.3
PC3  (via drill 0.3)
  Top 0.305: U1.26 33.88,20.35 v33.91,20.32
  Bottom 0.305: v33.91,20.32 37.21,20.32 45.85,11.68 55.75,11.68 58.42,9.02 PC.4
PC4/SDA  (via drill 0.3)
  Top 0.305: U1.27 34.35,21.15 v34.42,21.08 | v57.15,11.43 57.15,22.23 48.13,31.24 39.37,31.24 37.08,33.53 37.08,40.51 35.81,41.78 v32,41.78
  Bottom 0.305: v34.42,21.08 37.34,21.08 46.1,12.32 56.26,12.32 v57.15,11.43 60.96,7.62 PC.5 | J1.9 21.72,50.8 24.64,47.88 29.34,47.88 32,45.21 v32,41.78
PC5/SCL  (via drill 0.3)
  Top 0.305: U1.28 34.02,21.95 v34.04,21.97 | v57.91,11.94 57.91,22.86 48.9,31.88 39.62,31.88 37.85,33.66 37.85,41.15 36.45,42.55 v30.86,42.55
  Bottom 0.305: v34.04,21.97 37.34,21.97 46.35,12.95 56.9,12.95 v57.91,11.94 57.91,11.81 63.5,6.22 PC.6 | J1.10 19.3,50.8 23.11,46.99 28.7,46.99 30.86,44.83 v30.86,42.55
PD0/RX  (via drill 0.3)
  Top 0.305: U1.30 33.85,23.55 v33.91,23.5 | R2.1 19.05,40.51 19.05,44.2 21.84,46.99 50.29,46.99 v52.45,44.83
  Bottom 0.305: PD.1 63.25,50.8 61.34,48.9 59.69,48.9 56.9,46.1 | 56.9,46.1 53.72,46.1 v52.45,44.83 | v33.91,23.5 45.97,23.5 49.66,27.18 49.66,36.32 50.93,37.59 53.59,37.59 J7.3 55.88,38.99 57.28,40.39 57.28,45.72 56.9,46.1
PD1/TX  (via drill 0.3)
  Top 0.305: U1.31 34.26,24.35 v34.29,24.38 | R15.1 v14.99,40.39 | v20.45,46.86 21.21,47.62 50.8,47.62 v52.45,45.97
  Bottom 0.305: PD.2 60.33,50.8 56.39,46.86 53.34,46.86 v52.45,45.97 | v34.29,24.38 45.72,24.38 48.77,27.43 48.77,37.47 48.51,37.72 48.51,40.26 | v14.99,40.39 14.99,41.4 v20.45,46.86 | v52.45,45.97 52.26,45.78 | 48.51,40.26 48.51,42.04 v52.45,45.97 | J7.4 53.72,40.26 48.51,40.26
PD2/INT0  (via drill 0.3)
  Top 0.305: U1.32 v33.78,25.15
  Bottom 0.305: PD.3 55.24,47.62 53.09,47.62 47.88,42.42 47.88,27.69 45.34,25.15 v33.78,25.15
PD3/INT1  (via drill 0.3)
  Top 0.305: U1.1 32.99,26.64 v33.02,26.67
  Bottom 0.305: v33.02,26.67 45.85,26.67 47.24,28.07 47.24,42.8 52.83,48.39 54.74,48.39 55.88,49.53 PD.4
PD4  (via drill 0.3)
  Top 0.305: U1.2 29.61,27.58 29.84,27.81 31.88,27.81 v32.38,27.3
  Bottom 0.305: PD.5 53.34,50.16 46.61,43.43 46.61,28.7 45.21,27.3 v32.38,27.3
PD5  (via drill 0.3)
  Top 0.305: U1.9 v30.35,25.15
  Bottom 0.305: PD.6 45.85,45.85 45.85,29.34 44.45,27.94 31.88,27.94 30.35,26.42 v30.35,25.15
PD6  (via drill 0.3)
  Top 0.305: U1.10 29.56,24.35 v29.59,24.38
  Bottom 0.305: v29.59,24.38 29.59,26.54 31.62,28.57 43.81,28.57 45.09,29.84 45.09,47.62 PD.7
PD7  (via drill 0.3)
  Top 0.305: U1.11 28.89,23.55 v28.96,23.62 | J7.1 47.12,38.99 45.85,40.26 45.85,43.56 44.96,44.45 v44.07,44.45
  Bottom 0.305: v28.96,23.62 28.96,26.92 31.24,29.21 43.05,29.21 44.07,30.23 v44.07,44.45 44.07,49.15 PD.8
PWR_IN  (via drill 0.81)
  Top 0.61: R1.1 12.57,24.38 10.29,26.67 U2.3
  Top 0.762: 2.67,18.41 C1.+
  Top 0.813: v12.83,6.99 12.57,7.24 5.71,7.24 2.67,10.29 2.67,14.53 D1.- 2.74,18.34 C1.+ 2.79,18.92 v6.1,22.23 | v6.1,26.67 U2.3 | C6.+ 24.51,36.7 U4.3 v26.67,36.58 | D3.- 45.85,7.24 | 45.85,7.24 27.18,7.24 v27.05,7.37 | POWER.1 45.72,7.11 45.85,7.24
  Bottom 0.813: v6.1,22.23 v6.1,26.67 6.22,26.54 13.59,26.54 23.62,36.58 v26.67,36.58 | v27.05,7.37 13.21,7.37 v12.83,6.99
PWRKEY  (via drill 0.3)
  Top 0.305: v24.77,41.02 35.31,41.02 36.45,39.88 36.45,33.27 39.24,30.48 47.88,30.48 52.96,25.4 52.96,24.77 52.44,24.24 U6.8 | v4.06,44.96 2.22,44.96 KEY.2
  Bottom 0.305: v24.77,41.02 17.02,41.02 15.24,39.24 7.75,39.24 4.95,42.04 4.95,44.07 v4.06,44.96
RESET  (via drill 0.3)
  Top 0.305: ICSP.3 63.63,23.62 67.82,19.43 v67.82,18.67 | POWER.6 33.02,2.16 34.16,1.02 64.39,1.02 65.15,1.78 v65.15,3.68 | U1.29 33.13,22.75 v33.15,22.73 | C9.1 R11.2 17.14,41.78 14.99,43.94 7.62,43.94 6.99,44.58 6.99,48.77 8.76,50.55 RST.P$2
  Bottom 0.305: v33.15,22.73 33.15,14.1 | 33.15,14.1 33.15,2.67 POWER.6 | C9.1 24,40.39 24.38,40.01 31.75,40.01 32.64,39.12 32.64,35.69 31.62,34.67 28.32,34.67 22.1,28.45 22.1,16 24,14.1 33.15,14.1 | v65.15,3.68 64.26,4.57 64.26,6.73 67.82,10.29 v67.82,18.67
  other vias: 17.78,40.39
RST
  Top 0.305: D2.- 39.62,43.69 J5.1
RXD  (via drill 0.3)
  Top 0.305: 60.33,43.56 v60.2,43.56 60.21,43.55 U7.3 | U6.15 39.59,17.24 v44.07,21.72
  Bottom 0.305: v44.07,21.72 46.35,21.72 51.44,26.8 51.44,34.29 53.34,36.2 55.5,36.2 60.2,40.89 v60.2,43.56
RXD_5V
  Top 0.305: U7.12 54.47,43.55 J7.5
SIM_CLK  (via drill 0.3)
  Top 0.305: U6.31 53.26,13.41 52.45,14.22 v46.1,14.22
  Bottom 0.305: v46.1,14.22 R18.2
SIM_DATA  (via drill 0.3)
  Top 0.305: U6.30 52.26,12.51 51.44,13.34 45.97,13.34 45.09,14.22 45.09,14.86 45.85,15.62 v45.97,15.62
  Bottom 0.305: v45.97,15.62 R19.1
SIM_RST  (via drill 0.3)
  Top 0.305: U6.32 54.26,16.1 53.47,16.89 v45.97,16.89
  Bottom 0.305: v45.97,16.89 R17.2
SIM_VDD  (via drill 0.3)
  Top 0.305: v46.35,19.43 45.09,19.43 44.32,18.67 44.32,13.97 45.59,12.7 50.93,12.7 51.26,12.37 U6.29
  Bottom 0.305: U8.1 48.55,19.47 C24.1 v46.35,19.43
STATUS  (via drill 0.3)
  Top 0.305: v61.72,44.2 U7.4 | U6.49 54.58,29.24 v54.48,29.34
  Bottom 0.305: v54.48,29.34 59.56,34.42 59.56,36.58 61.72,38.73 v61.72,44.2
STATUS_5V
  Top 0.305: 12.95,44.83 R5.1 17.27,44.96 20.57,48.26 51.31,48.26 55.37,44.2 U7.11
TXD  (via drill 0.3)
  Top 0.305: 59.56,42.93 v59.44,42.93 59.47,42.9 U7.2 | U6.14 38.94,18.24 v43.18,22.48
  Bottom 0.305: v43.18,22.48 46.1,22.48 50.55,26.92 50.55,35.94 51.56,36.96 54.99,36.96 59.44,41.4 v59.44,42.93
TXD_5V
  Top 0.305: U7.13 54.58,42.9 53.72,42.04 53.72,40.26 J7.2
USB5V
  Top 0.305: R13.1 R14.1 1.4,33.02 1.78,33.4 3.81,33.4 4.83,34.42 4.83,40.51 5.84,41.53 9.14,41.53 9.65,42.04 11.81,42.04 F2.2
  Top 0.406: F2.2 14.48,41.66 16.13,41.66 16.89,40.89 16.89,38.1 16.63,37.84 U5.4 16.63,34.79 16,34.16 14.48,34.16 13.38,33.06 U5.20 13.38,28.28 13.84,27.81 15.37,27.81 16.26,26.92 Q1.3
VDD_EXT  (via drill 0.3)
  Top 0.305: U7.8 62.15,46.15 62.87,46.86 65.15,46.86 65.53,46.48 65.53,43.05 64.72,42.25 64.39,42.25 | 64.39,42.25 U7.1 63.93,42.25 | v64.26,41.66 64.26,42.12 64.39,42.25 | U6.7 51.59,25.24 v52.07,25.25
  Top 0.406: v62.48,21.59 R8.1
  Bottom 0.305: v64.26,41.66 64.26,37.85 61.85,35.43 61.85,33.91 63.37,32.38 66.67,32.38 67.82,31.24 67.82,25.15 66.8,24.13 62.48,24.13 | 62.48,24.13 v62.48,21.59 | 62.48,24.13 61.59,24.13 60.48,25.25 v52.07,25.25
VRTC
  Top 0.305: U6.17 C7.2
XTAL1
  Top 0.305: U1.7 25.61,28.24 R6.2 25.38,28.46 Y2.1
XTAL2
  Top 0.305: Y2.3 23.38,28.94 R6.1 24.81,27.51 U1.8

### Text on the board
tPlace: 1 | 1 | 1 | 1 | 9 | 8 | 7 | 6 | 5 | 4 | 3 | 2 | 1 | 0 | SCL | SDA | GND | 3 | 2 | 1 | 0 | RST | AREF | SIM_RX | SWserial | HWserial | SIM_TX | VCC | GND | - | + | IOREF | RST | 3V3 | 5V | GND | Vin | 0 | 1 | 2 | 3 | 4 | 5
bPlace: PIN | FUNCTION | RXD/PCINT16 | 0 | 1 | INT0 | TXD/PCINT17 | 2 | INT1/0C2B | 3 | PD[0:7] | XCK/T0 | 4 | 0C0B/T1 | 5 | 0C0A/AIN0 | 6 | AIN1 | 7 | ICP1 | 8 | Elecrow SIMduino | OC1A | 9 | SS/0C1B | 10 | UNO+SIM808 v1.0 | MOSI/OC2A | 11 | PB[0:5] | MISO | 12 | www.elecrow.com | SCK | 13 | ADC0 | 14 | ADC1 | 15 | ADC2 | 16 | PC[0:5] | ADC3 | 17 | ADC4/SDA | 18 | ADC5/SCL | 19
